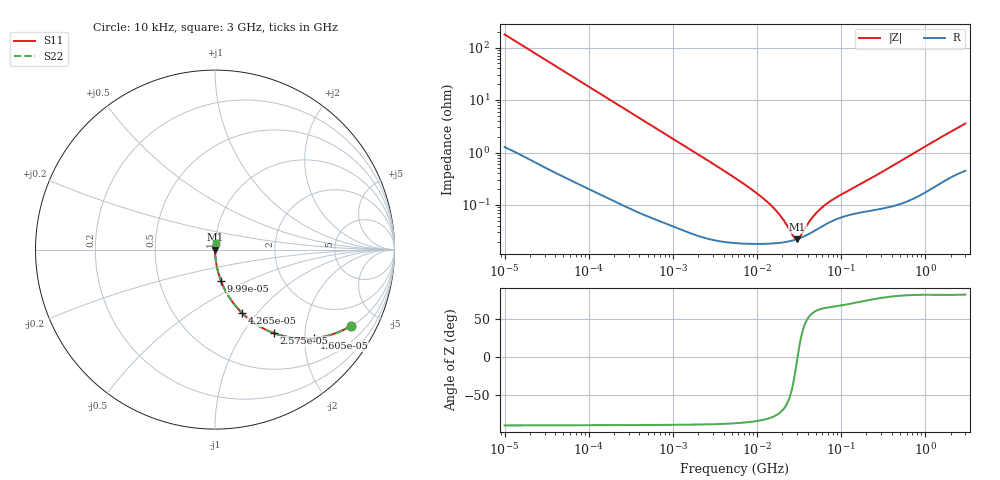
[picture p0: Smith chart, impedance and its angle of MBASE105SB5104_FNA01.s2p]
! MBASE105SB5104_FNA01  S-PARAMETER MODEL  ( Standard Model )
! Model Generated by TAIYO YUDEN Corporation (http://www.ty-top.com)
! Version 1.0
! TAIYO YUDEN Control No. 220601
! Copyright(c) 2013 TAIYO YUDEN CO.,LTD. All Rights Reserved.
! Product Description (link to TY-COMPAS)
! https://ds.yuden.co.jp/TYCOMPAS/or/detail?pn=MBASE105SB5104KFNA01&u=M
! Products Name : Multilayer Ceramic Capacitors
! Characteristics :
!  Capacitance : 0.1 [uF] , Rated Voltage : 16 [V] , TCC : X5R
!  Case Size : 1.0 x 0.5 / 0.039 x 0.02 [mm/inch] , Thickness : 0.5 / 0.02 [mm/inch]
!  (Conditions: Temperature = 25 [degC] , DC Bias Voltage = 0 [V])
! External Node Assignments :
!  1  o---| |---o  2
! GND o---------o GND
! Frequency Range : 10kHz  -  3GHz  [ 401 STEP ]
# MHZ S RI R 50
! Freq[MHz].  S11 Real  S11 Imag  S21 Real  S21 Imag  S12 Real  S12 Imag  S22 Real  S22 Imag
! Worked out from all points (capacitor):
!   401 points, 10 kHz to 3 GHz, reference 50 ohm
!   read as one part in series: C = 89.4 nF near 10.65 kHz
!   lowest |Z| = 22.3 mohm at 30.06 MHz (marker M1)
!   series resonance near 30.29 MHz, so ESL is about 310 pH
!   S11 on the Smith chart (normalised r, x): 10 kHz: 1.03, -3.55; 16.05 kHz: 1.02, -2.22; 25.75 kHz: 1.01, -1.39; 42.65 kHz: 1.01, -0.84; 99.9 kHz: 1.00, -0.36; 3 GHz: 1.01, +0.07
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0.01  0.7579 -0.4248  0.2421 0.4248  0.2421 0.4248  0.7579 -0.4248
0.016047  0.5516 -0.4934  0.4484 0.4934  0.4484 0.4934  0.5516 -0.4934
0.02575  0.3262 -0.4646  0.6738 0.4646  0.6738 0.4646  0.3262 -0.4646
0.042645  0.1522 -0.3546  0.8478 0.3546  0.8478 0.3546  0.1522 -0.3546
0.058452  0.0884 -0.2789  0.9116 0.2789  0.9116 0.2789  0.0884 -0.2789
0.082683  0.0472 -0.2067  0.9528 0.2067  0.9528 0.2067  0.0472 -0.2067
0.099902  0.0333 -0.1738  0.9667 0.1738  0.9667 0.1738  0.0333 -0.1738
0.226771  0.00739 -0.0792  0.9926 0.0792  0.9926 0.0792  0.00739 -0.0792
0.683653  0.00121 -0.0267  0.9988 0.0267  0.9988 0.0267  0.00121 -0.0267
5.477226  0.000198 -0.00327  0.9998 0.00327  0.9998 0.00327  0.000198 -0.00327
9.6612  0.000184 -0.00172  0.9998 0.00172  0.9998 0.00172  0.000184 -0.00172
14.55585  0.000185 -0.00098  0.9998 0.00098  0.9998 0.00098  0.000185 -0.00098
19.95104  0.000192 -0.000526  0.9998 0.000526  0.9998 0.000526  0.000192 -0.000526
27.34599  0.000213 -0.000125  0.9998 0.000125  0.9998 0.000125  0.000213 -0.000125
30.05882  0.000223 -9.12e-06  0.9998 9.12e-06  0.9998 9.12e-06  0.000223 -9.12e-06
33.04079  0.000236 0.000105  0.9998 -0.000105  0.9998 -0.000105  0.000236 0.000105
45.28751  0.000303 0.000485  0.9997 -0.000485  0.9997 -0.000485  0.000303 0.000485
58.28018  0.000385 0.000786  0.9996 -0.000786  0.9996 -0.000786  0.000385 0.000786
77.4027  0.000491 0.00113  0.9995 -0.00113  0.9995 -0.00113  0.000491 0.00113
374.4521  0.000937 0.00506  0.9991 -0.00506  0.9991 -0.00506  0.000937 0.00506
1321.625  0.00253 0.0168  0.9975 -0.0168  0.9975 -0.0168  0.00253 0.0168
3000  0.00569 0.035  0.9943 -0.035  0.9943 -0.035  0.00569 0.035
